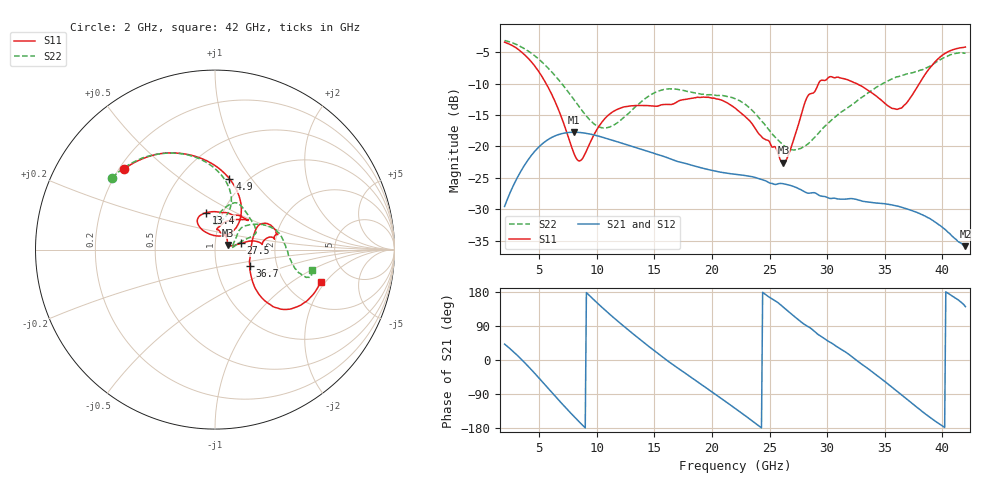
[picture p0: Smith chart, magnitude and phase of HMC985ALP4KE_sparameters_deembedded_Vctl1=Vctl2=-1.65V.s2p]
!s2p File: Measurements: S11, S21, S12, S22
# GHz S dB R 50.0
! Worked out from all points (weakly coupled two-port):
!   401 points, 2 GHz to 42 GHz, reference 50 ohm
!   highest |S21| = -17.73 dB at 8 GHz (marker M1); lowest = -35.9 dB at 42 GHz (marker M2)
!   lowest |S11| = -22.6 dB at 26.2 GHz (marker M3), VSWR 1.16, Z = 57.4 + j2.91 ohm
!   |S11| at or under -10 dB: 5.607 GHz to 29.25 GHz (23.64 GHz wide, 136 % of centre); 32.57 GHz to 37.99 GHz (5.417 GHz wide, 15.4 % of centre)
!   |S22| runs from -20.6 to -3.1 dB; largest |S21 - S12| = 0.00014
!   S11 on the Smith chart (normalised r, x): 2 GHz: 0.22, +0.36; 4.9 GHz: 0.84, +0.79; 13.4 GHz: 0.83, +0.36; 27.5 GHz: 1.33, +0.09; 36.7 GHz: 1.45, -0.27; 42 GHz: 3.10, -1.82
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2  -3.39 138.4  -29.56 41.9  -29.57 41.9  -3.12 145.0
3.4  -4.86 110.2  -23.99 3.4  -23.99 3.4  -4.10 121.7
4.9  -7.90 78.4  -20.21 -44.7  -20.22 -44.7  -5.99 97.9
6.2  -12.13 54.0  -18.46 -89.0  -18.47 -89.1  -8.35 80.6
8  -21.01 60.2  -17.73 -148.3  -17.74 -148.4  -12.48 69.8
8.7  -22.08 94.2  -17.81 -170.1  -17.82 -170.1  -14.23 71.9
10.7  -15.57 124.0  -18.64 132.2  -18.65 132.2  -17.06 90.3
13.4  -13.48 103.9  -20.18 62.8  -20.19 62.8  -13.61 82.4
15.4  -13.51 77.7  -21.36 15.3  -21.37 15.3  -11.15 69.1
18.9  -12.19 42.3  -23.32 -60.9  -23.33 -60.9  -11.60 43.2
22  -13.88 55.7  -24.42 -127.3  -24.43 -127.3  -12.39 21.1
24.5  -18.75 84.8  -25.37 176.3  -25.37 176.3  -16.32 16.6
26.2  -22.60 19.9  -25.95 139.2  -25.95 139.2  -19.81 7.8
27.5  -16.55 13.5  -26.71 106.2  -26.70 106.2  -20.45 8.1
28.7  -11.54 6.4  -27.38 80.8  -27.38 80.8  -18.96 20.1
29.5  -9.46 10.3  -27.92 62.0  -27.93 62.0  -17.37 29.6
31.1  -9.06 18.4  -28.39 30.5  -28.39 30.4  -14.70 39.3
33.3  -10.75 29.3  -28.80 -17.4  -28.80 -17.4  -11.83 33.2
35.4  -13.66 9.1  -29.26 -66.3  -29.27 -66.3  -9.47 21.6
36.7  -13.41 -24.5  -29.82 -98.0  -29.83 -98.0  -8.58 12.4
39.6  -6.12 -42.1  -32.35 -165.9  -32.34 -166.0  -6.45 -14.7
42  -4.16 -17.0  -35.89 140.9  -35.90 140.7  -5.13 -12.1
